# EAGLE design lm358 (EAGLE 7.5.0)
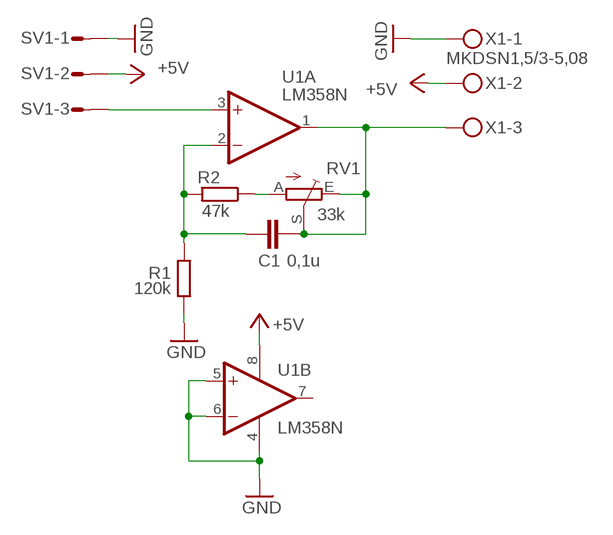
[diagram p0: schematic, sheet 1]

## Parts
C1  0,1u  C-EUC1206  [C1206]
R1  120k  R-EU_R1206  [R1206]
R2  47k  R-EU_R1206  [R1206]
RV1  33k  TRIM_EU-CA6V  [CA6V]
SV1  L03P  [L03P]
U1  LM358N  [DIL08]
X1  MKDSN1,5/3-5,08  [MKDSN1,5/3-5,08]

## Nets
+5V: SV1.2 U1.8(P:V+) X1.2
GND: R1.1 SV1.1 U1.4(P:V-) U1.5(B:+IN) U1.6(B:-IN) X1.1
N$1: SV1.3 U1.3(A:+IN)
N$2: C1.1 R1.2 R2.2 U1.2(A:-IN)
N$3: R2.1 RV1.A
N$4: C1.2 RV1.E RV1.S U1.1(A:OUT) X1.3
Unconnected: U1.7(B:OUT)

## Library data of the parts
C1 = rcl:C-EU: CAPACITOR, European symbol
R1 R2 = rcl:R-EU_: RESISTOR, European symbol
RV1 = pot:TRIM_EU-: POTENTIOMETER
SV1 = con-amp-mt:L03P: AMP MT CONNECTOR; OC_FARNELL: unknown; OC_NEWARK: unknown
U1 = linear:LM358: OP AMP also LM158; LM258; LM2904 Source: http://cache.national.com/ds/LM/LM158.pdf
X1 = con-phoenix-508:MKDSN1,5/3-5,08: MKDSN 1,5/ 3-5,08 Printklemme Nennstrom: 13,5 A Nennspannung: 250 V Rastermaß: 5,08 mm Polzahl: 3 Anschlussart: Schraubanschluss Montage: Löten Anschlussrichtung Leiter/Platine: 0 ° Artikelnummer: 1729131 Source: http://eshop.phoenixcontact.com .. 1729131.pdf

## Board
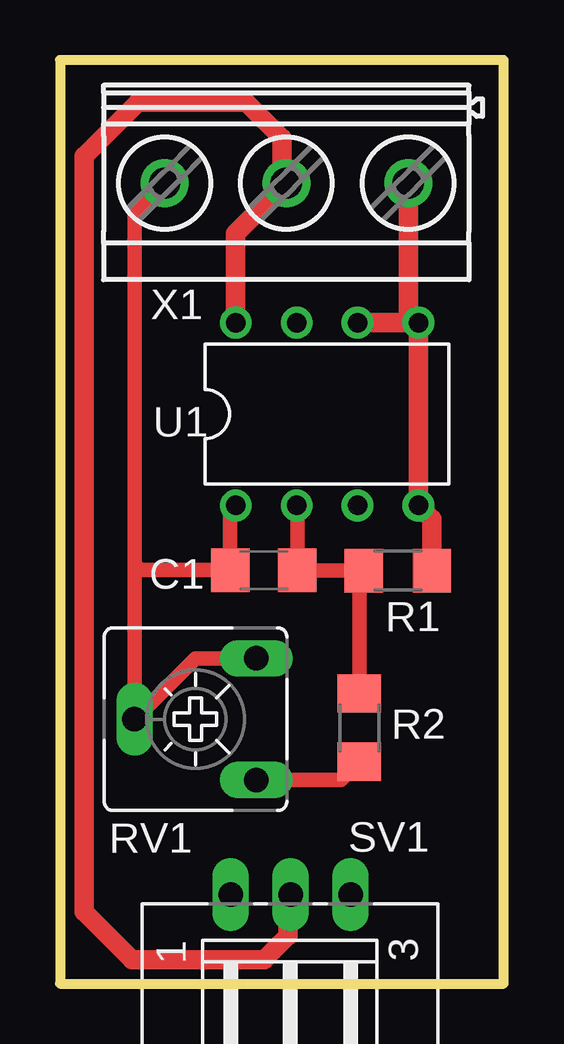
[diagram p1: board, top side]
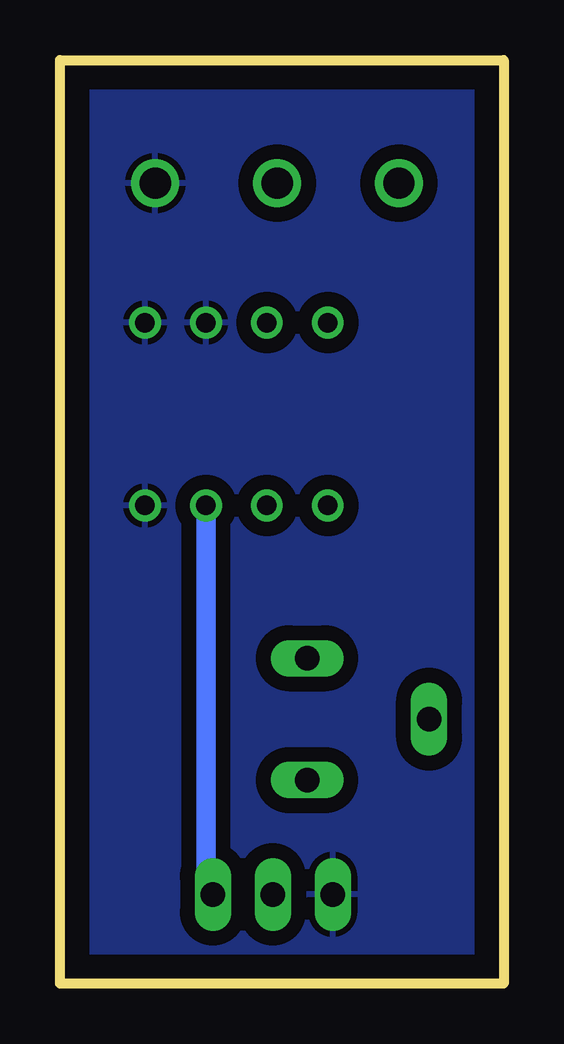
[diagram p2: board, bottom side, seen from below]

Size 18.5 x 38.5 mm. Coordinates in mm from the lower left corner, seen from the top.
Outline: 0,0 18.5,0 18.5,38.5 0,38.5 0,0
Copper layers (1*16): Top 0.035mm / dielectric 1.5mm / Bottom 0.035mm
Design rules "default": minimum track width 10mil, minimum drill 24mil, track to track 8mil, track to pad 8mil, pad to pad 8mil, via to via 8mil, smd to smd 8mil, copper to edge 40mil, drill to drill 8mil, minimum pad ring 10mil, minimum via ring 8mil, stop-mask expansion 4mil, vias tented up to drill 0mil, thermal gap 10mil

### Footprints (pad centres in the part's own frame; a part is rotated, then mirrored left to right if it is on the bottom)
C1206 = smd 1.6 x 1.8: 1 -1.4,0; 2 1.4,0
R1206 = smd 1.6 x 1.803: 1 -1.422,0; 2 1.422,0
CA6V = drill 1.016 long: A -2.54,-2.54; E 2.54,-2.54; S 0,2.54
L03P = drill 1.016 long: 1 2.5,-6.25; 2 0,-6.25; 3 -2.5,-6.25
DIL08 = drill 0.813 pad 1.27: 1 -3.81,-3.81; 2 -1.27,-3.81; 3 1.27,-3.81; 4 3.81,-3.81; 5 3.81,3.81; 6 1.27,3.81; 7 -1.27,3.81; 8 -3.81,3.81
MKDSN1,5/3-5,08 = drill 1.3 pad 2: 1 -7.641,0.025; 2 -2.561,0.025; 3 2.519,0.025

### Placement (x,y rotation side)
C1  8.5,17.23 180 top
R1  14.09,17.21 180 top
R2  12.48,10.67 90 top
RV1  5.65,11.02 90 top
SV1  9.62,-2.54 180 top
U1  11.14,23.74 0 top
X1  6.88,33.39 180 top

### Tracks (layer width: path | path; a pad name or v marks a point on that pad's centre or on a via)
+5V
  Top 0.813: U1.8 7.33,31.25 X1.2 9.25,33.56 9.25,35.25 7.75,36.75 3.25,36.75 1,34.5 1,3 3,1 8.5,1 9.5,2 9.5,3.59 SV1.2
GND
  Top 0.813: R1.1 15.51,19.37 U1.4 U1.5 | U1.6 U1.5 | X1.1 14.52,27.98 U1.5
  pour Bottom (isolate 0.61): 0.25,38.5 19.25,38.5 19.25,0 0.25,0
N$1
  Bottom 0.813: U1.3 12.41,4 SV1.3
N$2
  Top 0.61: R2.2 12.48,17.02 R1.2 9.92,17.21 C1.1 9.9,19.9 U1.2
N$3
  Top 0.61: RV1.A 11.71,8.48 R2.1
N$4
  Top 0.61: 3.11,17.5 RV1.S 5.65,13.56 RV1.E | 3.11,17.5 3.11,32.11 X1.3 | 3.11,17.5 3.38,17.23 C1.2 7.1,19.7 U1.1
